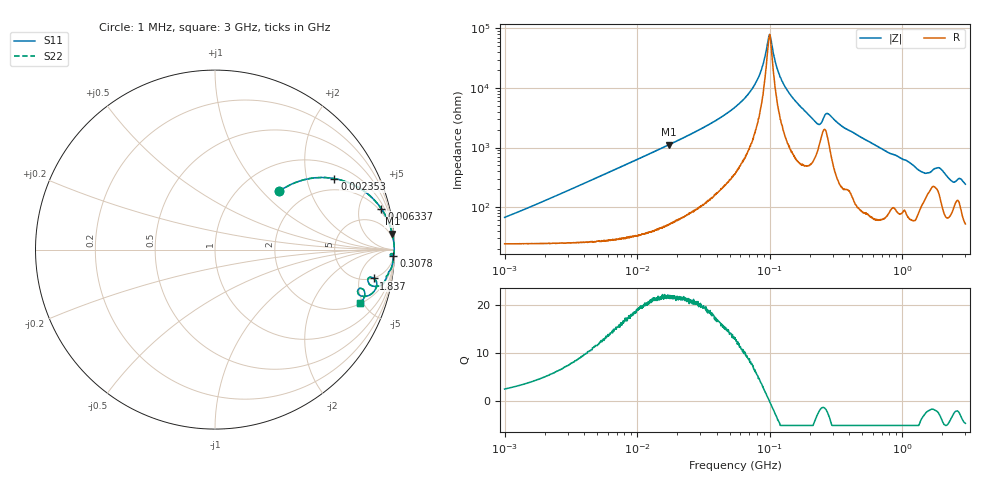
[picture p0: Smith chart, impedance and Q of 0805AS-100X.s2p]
!s-Parameter Generated by FASTRON Sdn. Bhd.
!FASTRON P/N : 0805AS-100X
!Keysight Technologies: E4991B_MY54100416_A.01.15
!Date: Mon Jun 15 13:00:24 2026
!Version  :Rev01  Mon Jun 15 13:00:24 2026
!Data & Calibration Information:
!Freq  S11  S21  S12  S22
!PortZ  Port1:50+j0  Port2:50+j0
!When reading reference impedance value at option line is always used.
! Remarks : This data is being provided solely for informational purposes.
# Hz S dB R 50
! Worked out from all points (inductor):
!   1601 points, 1 MHz to 3 GHz, reference 50 ohm
!   read as one part in series: L = 9.97 uH near 1.156 MHz
!   highest Q = 22 at 17.33 MHz (marker M1), where L = 10.2 uH
!   self-resonance near 99.35 MHz
!   S11 on the Smith chart (normalised r, x): 1 MHz: 1.48, +1.25; 2.353 MHz: 1.50, +2.95; 6.337 MHz: 1.56, +7.96; 307.8 MHz: 9, -58; 1.837 GHz: 4.91, -8.19; 3 GHz: 2.04, -4.74
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1000000  -6.32 42.1  -2.87 -26.8  -2.87 -26.8  -6.32 42.1
2352975  -2.23 30.7  -5.71 -49.8  -5.71 -49.8  -2.23 30.7
3804036  -1.01 21.7  -8.60 -62.2  -8.60 -62.2  -1.01 21.7
6337400  -0.41 13.8  -12.40 -72.2  -12.40 -72.2  -0.41 13.8
1.447069e7  -0.09 6.2  -19.40 -81.2  -19.40 -81.2  -0.09 6.2
1.732704e7  -0.07 5.1  -21.00 -82.3  -21.00 -82.3  -0.07 5.1
5.504702e7  -0.02 1.2  -33.60 -84.4  -33.60 -84.4  -0.02 1.2
7.971695e7  -0.01 0.4  -42.30 -79.7  -42.30 -79.7  -0.01 0.4
8.723049e7  -0.01 0.3  -46.60 -74.3  -46.60 -74.3  -0.01 0.3
9.984923e7  -0.01 -0.0  -58.00 0.8  -58.00 0.8  -0.01 -0.0
1.142934e8  -0.01 -0.3  -46.40 74.1  -46.40 74.1  -0.01 -0.3
1.282345e8  -0.01 -0.5  -41.10 80.5  -41.10 80.5  -0.01 -0.5
2.083556e8  -0.05 -1.8  -29.90 78.1  -29.90 78.1  -0.05 -1.8
2.373059e8  -0.17 -2.0  -27.90 60.6  -27.90 60.6  -0.17 -2.0
2.729971e8  -0.10 -1.4  -31.50 64.7  -31.50 64.7  -0.10 -1.4
3.078328e8  -0.05 -1.9  -29.40 79.7  -29.40 79.7  -0.05 -1.9
7.925923e8  -0.16 -6.9  -18.40 77.6  -18.40 77.6  -0.16 -6.9
1.423359e9  -0.85 -13.0  -12.60 60.2  -12.60 60.2  -0.85 -13.0
1.837163e9  -0.93 -10.3  -14.10 54.1  -14.10 54.1  -0.93 -10.3
2.335937e9  -1.20 -17.4  -10.10 57.0  -10.10 57.0  -1.20 -17.4
2.700748e9  -1.34 -15.1  -11.00 52.3  -11.00 52.3  -1.34 -15.1
3e9  -1.29 -20.3  -8.99 57.3  -8.99 57.3  -1.29 -20.3
